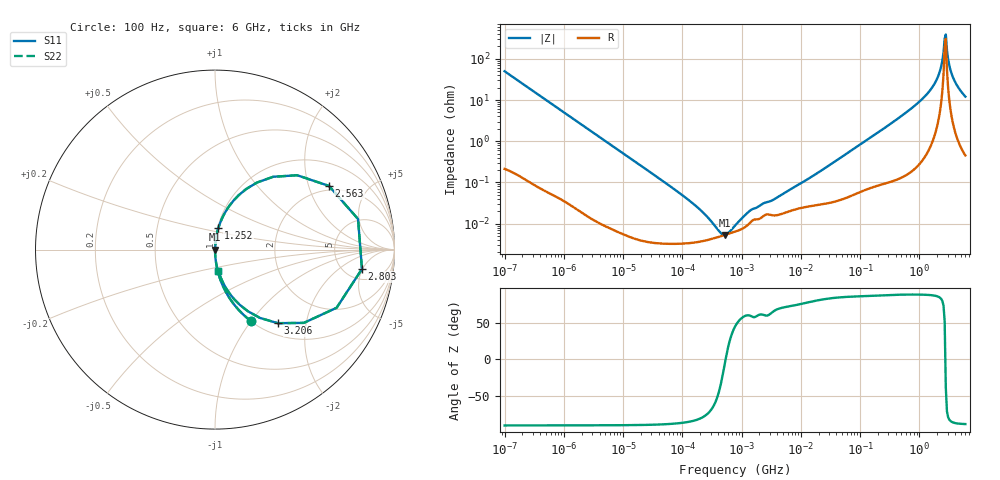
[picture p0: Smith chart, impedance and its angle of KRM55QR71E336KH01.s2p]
!Murata Part Number: KRM55QR71E336KH01
!These Parameters are Measured in Series Mode Connection
!Data Generated on Jan 08, 2026
!  o--ll--o
!Port1  Port2
!  o------o
!Operation Temp=25[degC], DC Bias Voltage=0[V]
!Freq. Start=100[Hz] Stop=6[GHz] 401[Steps]
# Hz S RI R 50
!Freq.(Hz) S11(Real) S11(Imag) S21(Real) S21(Imag) S12(Real) S12(Imag) S22(Real) S22(Imag)
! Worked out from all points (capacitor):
!   401 points, 100 Hz to 6 GHz, reference 50 ohm
!   read as one part in series: C = 31.7 uF near 109 Hz
!   lowest |Z| = 5.33 mohm at 517.7 kHz (marker M1)
!   series resonance near 537.4 kHz, so ESL is about 2.8 nH
!   S11 on the Smith chart (normalised r, x): 100 Hz: 1.00, -1.00; 1.252 GHz: 1.01, +0.25; 2.563 GHz: 1.82, +2.74; 2.803 GHz: 7.14, -4.86; 3.206 GHz: 1.20, -1.39; 6 GHz: 1.01, -0.24
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100  0.2022 -0.3995  0.7978 0.3995  0.7978 0.3995  0.2022 -0.3995
383  0.0177 -0.1292  0.9823 0.1292  0.9823 0.1292  0.0177 -0.1292
2008  0.000823 -0.0253  0.9992 0.0253  0.9992 0.0253  0.000823 -0.0253
40335  3.48e-05 -0.00126  1 0.00126  1 0.00126  3.48e-05 -0.00126
147774  3.44e-05 -0.000316  1 0.000316  1 0.000316  3.44e-05 -0.000316
330837  4.36e-05 -9.07e-05  1 9.07e-05  1 9.07e-05  4.36e-05 -9.07e-05
517687  5.29e-05 -6.4e-06  0.9999 6.4e-06  0.9999 6.4e-06  5.29e-05 -6.4e-06
774597  6.38e-05 6.3e-05  0.9999 -6.3e-05  0.9999 -6.3e-05  6.38e-05 6.3e-05
1449809  0.000112 0.000186  0.9999 -0.000186  0.9999 -0.000186  0.000112 0.000186
3394479  0.000159 0.000342  0.9998 -0.000342  0.9998 -0.000342  0.000159 0.000342
1.555665e7  0.000272 0.00138  0.9997 -0.00138  0.9997 -0.00138  0.000272 0.00138
3.124326e8  0.00165 0.0253  0.9983 -0.0253  0.9983 -0.0253  0.00165 0.0253
1.251881e9  0.0193 0.1217  0.9807 -0.1217  0.9807 -0.1217  0.0193 0.1217
2.048624e9  0.132 0.303  0.868 -0.303  0.868 -0.303  0.132 0.303
2.34314e9  0.3244 0.4058  0.6756 -0.4058  0.6756 -0.4058  0.3244 0.4058
2.562649e9  0.6347 0.3549  0.3653 -0.3549  0.3653 -0.3549  0.6347 0.3549
2.802721e9  0.8188 -0.1081  0.1812 0.1081  0.1812 0.1081  0.8188 -0.1081
3.065283e9  0.4947 -0.4083  0.5053 0.4083  0.5053 0.4083  0.4947 -0.4083
3.205649e9  0.3493 -0.41  0.6507 0.41  0.6507 0.41  0.3493 -0.41
3.505958e9  0.1831 -0.3433  0.8169 0.3433  0.8169 0.3433  0.1831 -0.3433
3.8344e9  0.107 -0.2765  0.893 0.2765  0.893 0.2765  0.107 -0.2765
6e9  0.0188 -0.1184  0.9812 0.1184  0.9812 0.1184  0.0188 -0.1184
